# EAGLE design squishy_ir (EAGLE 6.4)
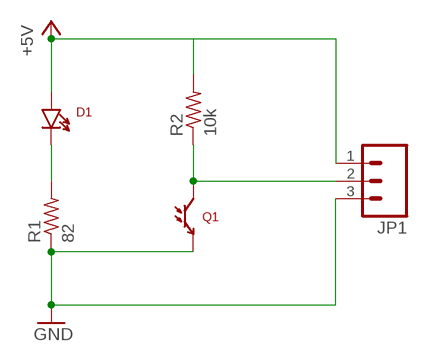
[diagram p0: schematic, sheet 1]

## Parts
D1  LTE-302  [LTE-302]
JP1  M03  [JST-3-SMD]
Q1  LTR-301  [LTR-301]
R1  82  R-US_0204/7  [0204/7]
R2  10k  R-US_0204/7  [0204/7]

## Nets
+5V: D1.A JP1.1 R2.2
GND: JP1.3 Q1.E R1.1
N$1: D1.C R1.2
N$2: JP1.2 Q1.C R2.1

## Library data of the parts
D1 = SparkFun-LED:LTE-302: Through-hole side-firing 940nm IR LED
JP1 = SparkFun-Connectors:M03: Header 3 Standard 3-pin 0.1" header. Use with straight break away headers (SKU : PRT-00116), right angle break away headers (PRT-00553), swiss pins (PRT-00743), machine pins (PRT-00117), and female headers (PRT-00115). Molex polarized connector foot print use with SKU : PRT-08232 with associated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
Q1 = SparkFun-Sensors:LTR-301: Through-hole side-receiving IR phototransistor
R1 R2 = resistor:R-US_: RESISTOR, American symbol

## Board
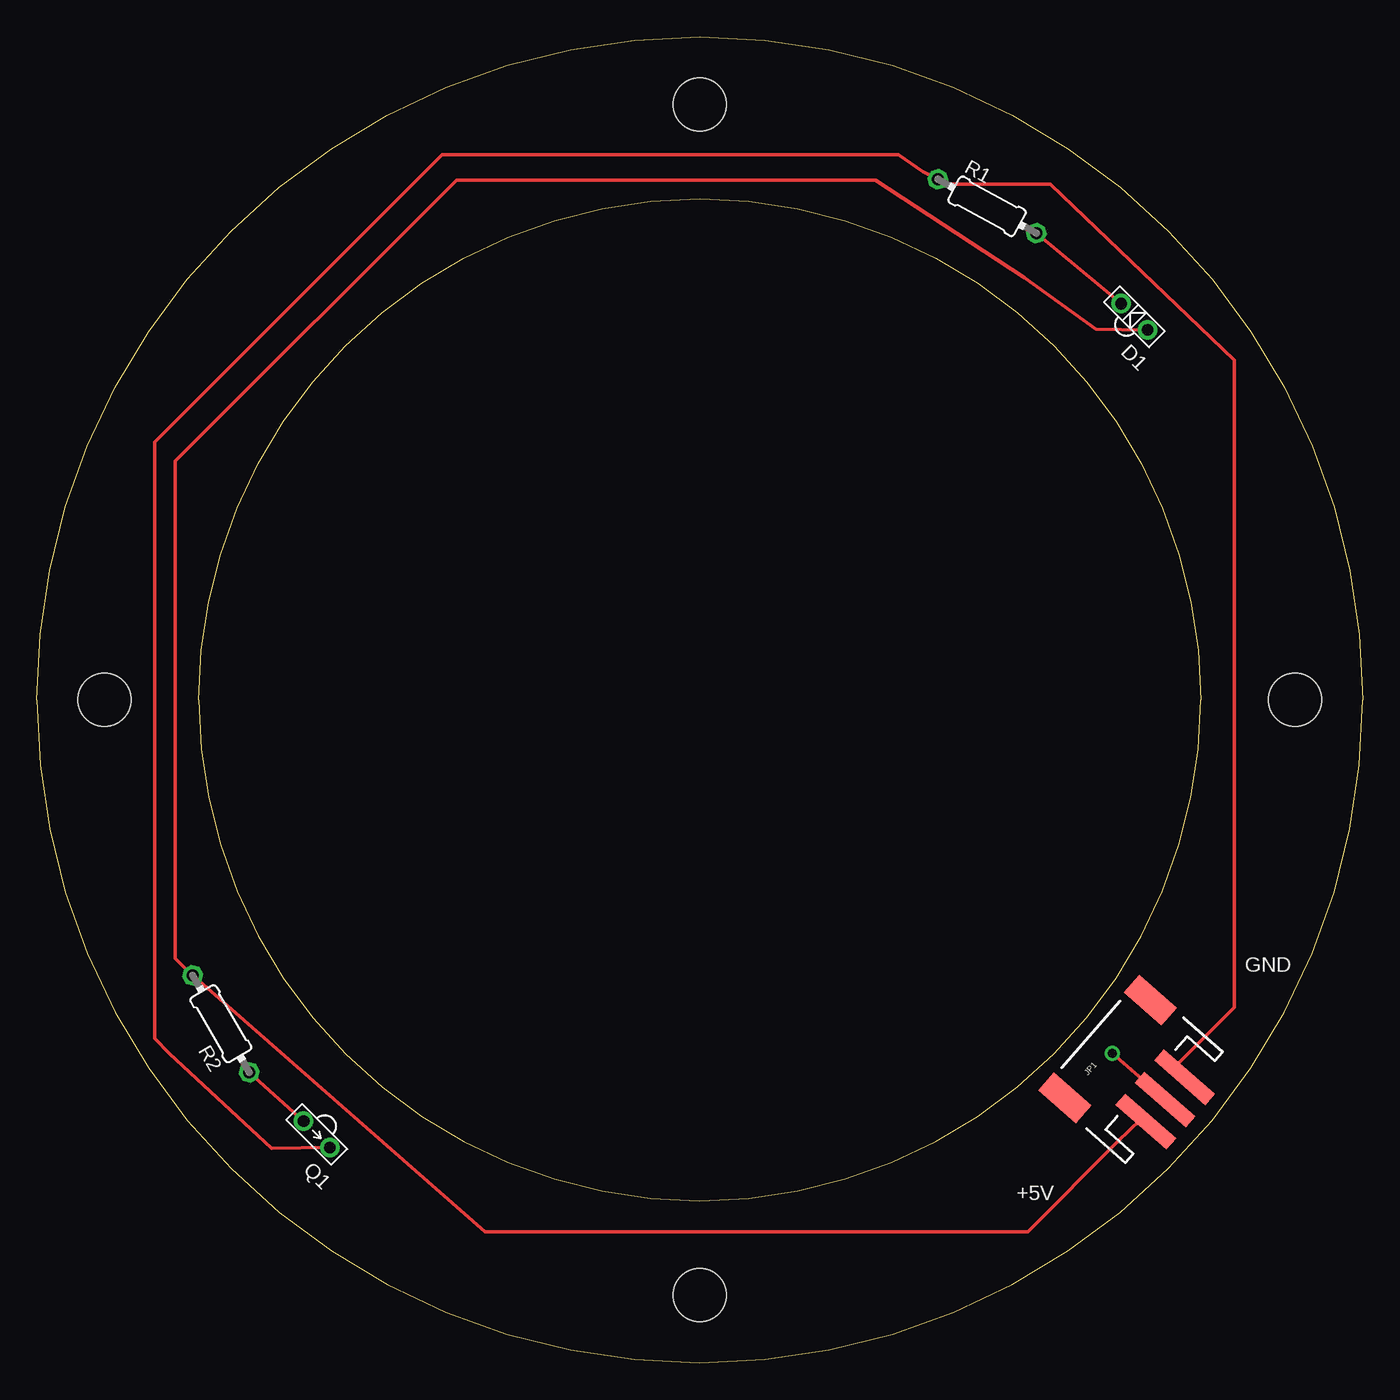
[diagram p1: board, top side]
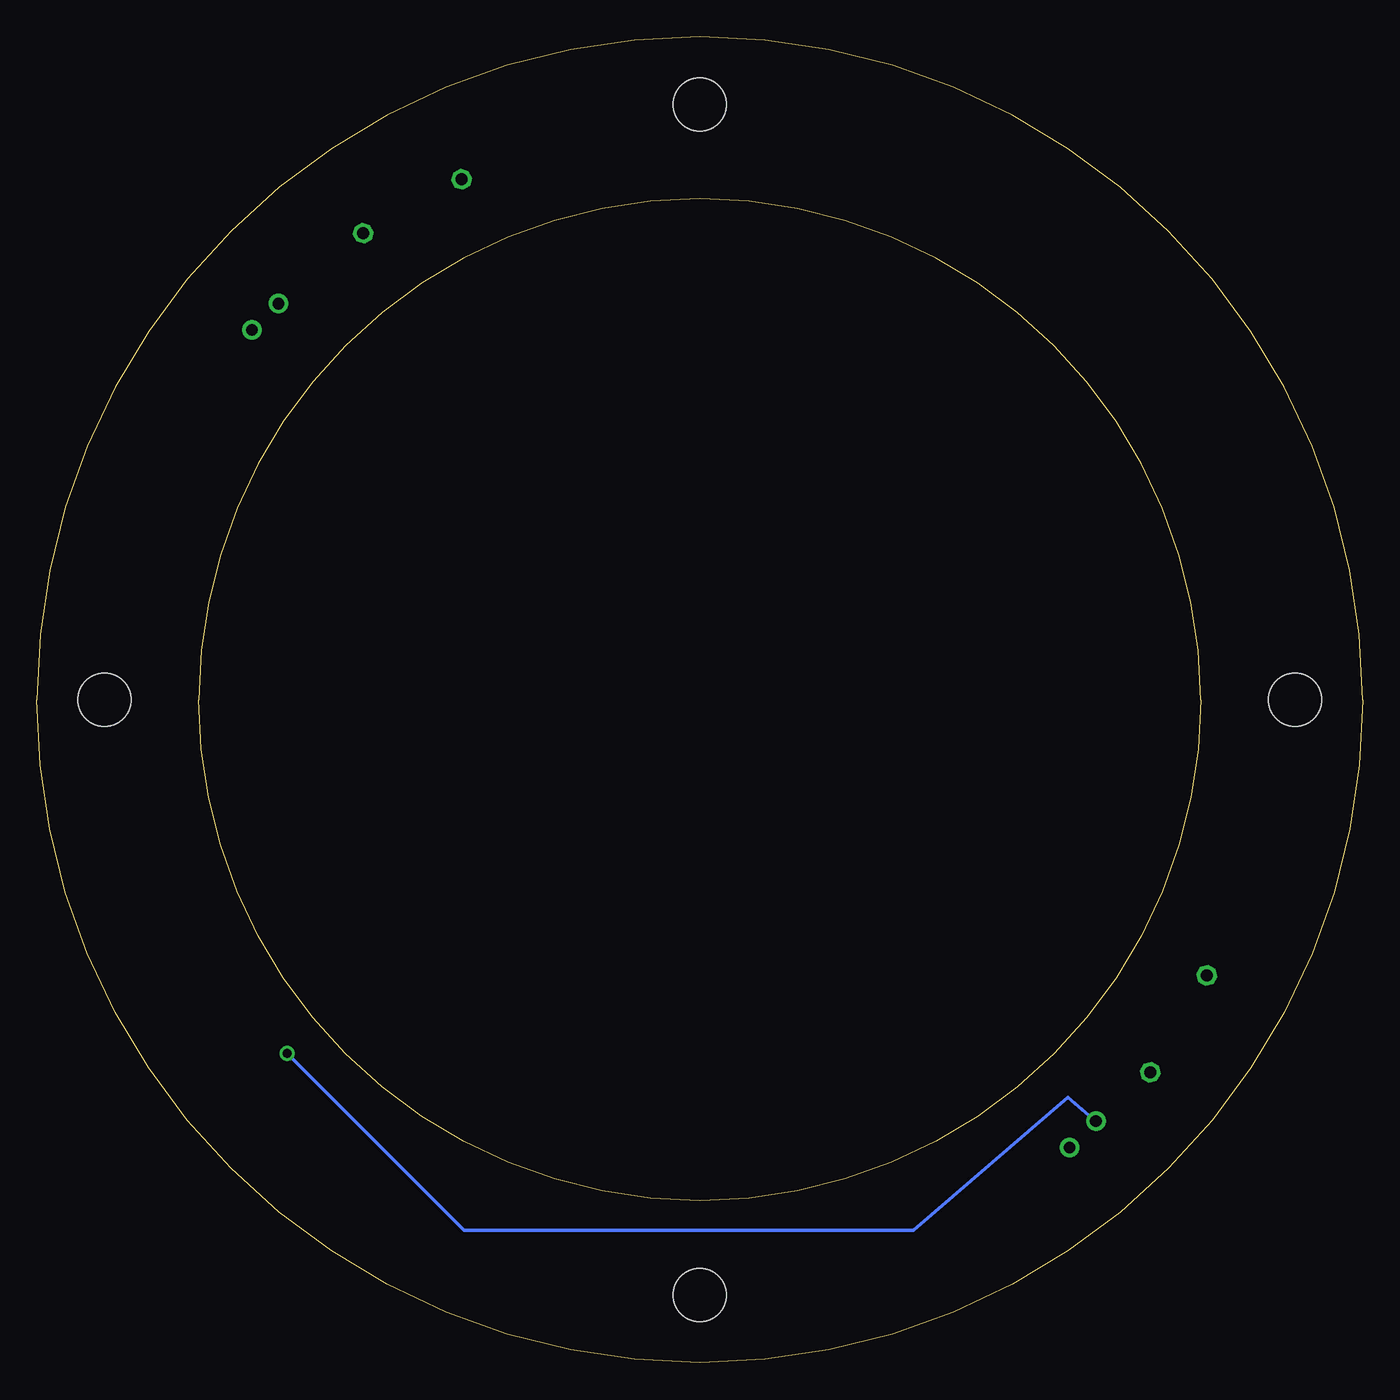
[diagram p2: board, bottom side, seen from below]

Size 90 x 90 mm. Coordinates in mm from the lower left corner, seen from the top.
Outline: 0,45 arc-180 90,45 arc-180 0,45
Outline: 11,45 arc-180 79,45 arc-180 11,45
Copper layers (1*16): Top 0.035mm / dielectric 1.5mm / Bottom 0.035mm
Design rules "default": minimum track width 10mil, minimum drill 24mil, track to track 8mil, track to pad 8mil, pad to pad 8mil, via to via 8mil, smd to smd 8mil, copper to edge 40mil, drill to drill 8mil, minimum pad ring 10mil, minimum via ring 8mil, stop-mask expansion 4mil, vias tented up to drill 0mil, thermal gap 10mil
Holes 3.6 mm at 45,85.4 4.6,45 85.4,45 45,4.6

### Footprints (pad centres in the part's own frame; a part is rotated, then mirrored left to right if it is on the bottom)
LTE-302 = drill 0.8: A 1.27,0; C -1.27,0
JST-3-SMD = smd 1 x 4.6: 1 -1.99,-4.77; 2 0.01,-4.77; 3 2.01,-4.77 | smd 1.6 x 3.4: NC1 -4.39,0.43; NC2 4.41,0.43
LTR-301 = drill 0.8: C 1.27,0; E -1.27,0
0204/7 = drill 0.813 octagon: 1 -3.81,0; 2 3.81,0

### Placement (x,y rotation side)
D1  74.5,71 315 top
JP1  73,21 48.8 top
Q1  19,15.5 135 top
R1  64.5,78.5 331.3 top
R2  12.5,23 120.3 top

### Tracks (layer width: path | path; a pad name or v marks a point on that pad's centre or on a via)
+5V
  Top 0.254: 10.16,26.67 9.39,27.44 9.39,61.19 28.48,80.28 56.92,80.28 67.04,73.66 71.89,70.16 D1.A | 10.16,26.67 30.44,8.89 67.27,8.89 73.39,15.01 74.93,16.51 JP1.1 | 10.16,26.67 R2.2
GND
  Top 0.254: JP1.3 77.47,20.32 81.28,24.13 81.28,68.04 68.81,80.01 60.96,80.01 R1.1 60.16,80.84 58.5,82 27.5,82 8,62.5 8,22 9,21 15.96,14.54 Q1.E
N$1
  Top 0.254: R1.2 D1.C
N$2  (via drill 0.6)
  Top 0.254: R2.1 Q1.C | JP1.2 v73,21
  Bottom 0.254: v73,21 61,9 30.5,9 20,18 Q1.C

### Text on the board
tPlace: D1 | GND | Q1 | +5V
